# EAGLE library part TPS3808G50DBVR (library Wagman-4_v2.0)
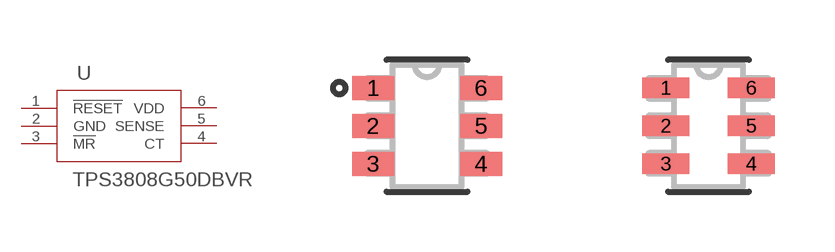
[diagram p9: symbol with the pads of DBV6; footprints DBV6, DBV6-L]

Designator prefix U

## TPS3808G50DBVR (MANUFACTURER_PART_NUMBER: TPS3808G50DBVR; VENDOR: Texas Instruments)  [DBV6]
1  !RESET  pas
2  GND  pwr
3  !MR  pas
4  CT  pas
5  SENSE  pas
6  VDD  pwr

## TPS3808G50DBVRDBV6-L (MANUFACTURER_PART_NUMBER: TPS3808G50DBVR; VENDOR: Texas Instruments)  [DBV6-L]
Pads as for DBV6

## TPS3808G50DBVRDBV6-M (MANUFACTURER_PART_NUMBER: TPS3808G50DBVR; VENDOR: Texas Instruments)  [DBV6-M]
Pads as for DBV6

## Footprint DBV6 (pad centres in mm)
smd 1.05 x 0.6: 1 -1.35,0.95; 2 -1.35,0; 3 -1.35,-0.95; 4 1.35,-0.95; 5 1.35,0; 6 1.35,0.95

## Footprint DBV6-L (pad centres in mm)
smd 1.168 x 0.508: 1 -1.067,0.95; 2 -1.067,0; 3 -1.067,-0.95; 4 1.067,-0.95; 5 1.067,0; 6 1.067,0.95

## Footprint DBV6-M (pad centres in mm)
smd 1.778 x 0.61: 1 -1.168,0.95; 2 -1.168,0; 3 -1.168,-0.95; 4 1.168,-0.95; 5 1.168,0; 6 1.168,0.95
